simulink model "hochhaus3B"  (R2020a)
settings: Solver=ode45  StartTime=0.0  StopTime=5  MaxStep=1e-2  RelTol=1e-3  EnableMultiTasking=on

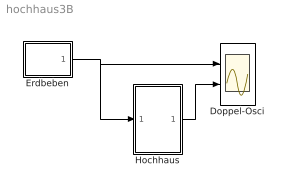
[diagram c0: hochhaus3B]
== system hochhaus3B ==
  Doppel-Osci : Scope  NumInputPorts=2
  Erdbeben : Subsystem  mask(Erdbeben){Fmax=1e3, Omega=10, Tab=0.9, Frausch=100}
      mask prompts: Fmax "Kraftamplitude"; Omega "Kreisfrequenz"; Tab "Abklingzeit"; Frausch "Rauschamplitude"
      mask help: Anregung durch Erdbebenwelle
  Hochhaus : Subsystem  mask(Schwingerkette){m=[6,6,1]*1e3, c=[3,3,1]*1e6, x0=0, v0=0}
      mask prompts: m "Massen"; c "Steifigkeiten"; x0 "Anfangsauslenkungen"; v0 "Anfangsgeschwindigkeiten"
      mask help: eindimensionale Schwingerkette mit oberem freien Ende und Krafterregung am Fusspunkt
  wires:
  Erdbeben/1(F) -> Doppel-Osci/1, Hochhaus/1(F)
  Hochhaus/1(x) -> Doppel-Osci/2

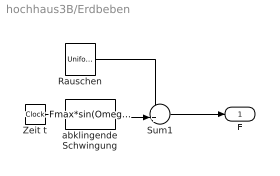
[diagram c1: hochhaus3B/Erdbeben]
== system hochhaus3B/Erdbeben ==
  Rauschen : UniformRandomNumber  Minimum=-Frausch  Maximum=Frausch  SampleTime=0
  Sum1 : Sum  Inputs=++|  InputSameDT=on  SaturateOnIntegerOverflow=on
  Zeit t : Clock
  abklingende Schwingung : Fcn  Expr=Fmax*sin(Omega*u[1])*exp(-u[1]/Tab)
  F : Outport
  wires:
  Zeit t/1 -> abklingende Schwingung/1
  abklingende Schwingung/1 -> Sum1/2
  Rauschen/1 -> Sum1/1
  Sum1/1 -> F/1

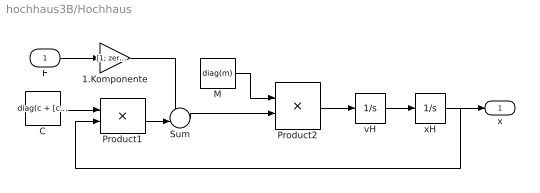
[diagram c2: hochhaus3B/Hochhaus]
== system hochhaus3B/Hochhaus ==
  F : Inport
  1.Komponente : Gain  Gain=[1; zeros(length(m)-1,1)]  SaturateOnIntegerOverflow=on
  C : Constant  Value=diag(c + [c(2:end),0]) - diag(c(2:end),1) - diag(c(2:end),-1)  VectorParams1D=off
  M : Constant  Value=diag(m)  VectorParams1D=off
  Product1 : Product  Multiplication=Matrix(*)  InputSameDT=on  SaturateOnIntegerOverflow=on
  Product2 : Product  Inputs=/*  Multiplication=Matrix(*)  InputSameDT=on  SaturateOnIntegerOverflow=on
  Sum : Sum  Inputs=+-|  InputSameDT=on  SaturateOnIntegerOverflow=on
  vH : Integrator  InitialCondition=v0
  xH : Integrator  InitialCondition=x0
  x : Outport
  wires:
  1.Komponente/1 -> Sum/1
  F/1 -> 1.Komponente/1
  M/1 -> Product2/1
  Product2/1 -> vH/1
  Sum/1 -> Product2/2
  C/1 -> Product1/1
  Product1/1 -> Sum/2
  xH/1 -> x/1, Product1/2
  vH/1 -> xH/1
